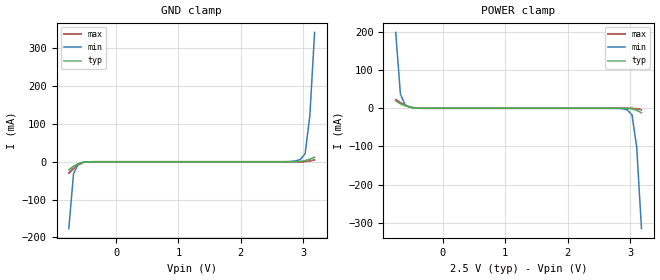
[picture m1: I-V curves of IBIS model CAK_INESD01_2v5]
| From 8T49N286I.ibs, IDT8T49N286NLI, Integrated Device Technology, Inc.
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| 4.00000e+00   -1.39435e-02   -4.76170e-01   -2.47919e-03
| 4.10000e+00   -3.14988e-02   -7.57889e-01   -1.14633e-02
| 4.20000e+00   -2.28002e-01   -1.04024e+00   -2.64916e-02
| 4.30000e+00   -6.05524e-01   -1.32301e+00   -4.21848e-02
| 4.40000e+00   -9.83643e-01   -1.60614e+00   -8.92880e-02
| 4.50000e+00   -1.36229e+00   -1.88958e+00   -5.31426e-01
| 4.60000e+00   -1.74142e+00   -2.17332e+00   -1.01589e+00
| 4.70000e+00   -2.12097e+00   -2.45733e+00   -1.50090e+00
| 4.80000e+00   -2.50090e+00   -2.74162e+00   -1.98635e+00
| 4.90000e+00   -2.88116e+00   -3.02615e+00   -2.47218e+00
| 5.00000e+00   -3.26171e+00   -3.31092e+00   -2.95830e+00
| 5.10000e+00   -3.64251e+00   -3.59590e+00   -3.44467e+00
| 5.20000e+00   -4.02353e+00   -3.88109e+00   -3.93123e+00
| 5.30000e+00   -4.40474e+00   -4.16647e+00   -4.41796e+00
| 5.40000e+00   -4.78610e+00   -4.45202e+00   -4.90484e+00
| 5.50000e+00   -5.16760e+00   -4.73774e+00   -5.39184e+00
| 5.60000e+00   -5.54921e+00   -5.02360e+00   -5.87893e+00
| 5.70000e+00   -5.93093e+00   -5.30959e+00   -6.36610e+00
| 5.80000e+00   -6.31272e+00   -5.59572e+00   -6.85331e+00
| 5.90000e+00   -6.69459e+00   -5.88196e+00   -7.34056e+00
| 6.00000e+00   -7.07651e+00   -6.16831e+00   -7.82783e+00
| 6.10000e+00   -7.45848e+00   -6.45476e+00   -8.31510e+00
| 6.20000e+00   -7.84049e+00   -6.74131e+00   -8.80238e+00
| 6.30000e+00   -8.22253e+00   -7.02794e+00   -9.28965e+00
| 6.40000e+00   -8.60459e+00   -7.31465e+00   -9.77691e+00
| 6.50000e+00   -8.98667e+00   -7.60144e+00   -1.02642e+01
| 6.60000e+00   -9.36876e+00   -7.88830e+00   -1.07514e+01
[Model]   CAK_INESD01_2v5
Model_type   Input
Polarity   Non-Inverting
Vinl = 0.7V
Vinh = 1.7V
|   typ   min   max
C_comp   2pF   1.5pF   2.5pF
|   typ   min   max
[Voltage range]   2.5V   2.375V   2.625V
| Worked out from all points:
|   GND clamp passes 1 mA (typ) near -0.50 V on its own axis
|   POWER clamp passes 1 mA (typ) near -0.46 V on its own axis
[GND_clamp]
|Voltage   I (typ)   I (min)   I (max)
|Note, modeling breaks down at 250mA and above.  This is well beyond the functional   |
|operating range of the device.  Should this scenario occur, catastrophic failure and   |
|possible damage to the device and/or board is of higher concern than the I-V curve   |
|behavior.  The IBIS checker will flag currents in excess of 10A with warnings.  Lines   |
|with currents in excess of 0.35 A have been commented out.  The points still remain|
|available to the user if the user desires to use them.   |
|-2.50000e+00   -6.31272e+00   -5.12654e+00   -7.65728e+00
|-2.42424e+00   -6.02348e+00   -4.90993e+00   -7.28814e+00
|-2.34848e+00   -5.73428e+00   -4.69340e+00   -6.91901e+00
|-2.27273e+00   -5.44513e+00   -4.47695e+00   -6.54991e+00
|-2.19697e+00   -5.15604e+00   -4.26060e+00   -6.18082e+00
|-2.12121e+00   -4.86701e+00   -4.04434e+00   -5.81177e+00
|-2.04545e+00   -4.57807e+00   -3.82819e+00   -5.44276e+00
|-1.96970e+00   -4.28920e+00   -3.61215e+00   -5.07380e+00
|-1.89394e+00   -4.00043e+00   -3.39622e+00   -4.70491e+00
|-1.81818e+00   -3.71177e+00   -3.18041e+00   -4.33609e+00
|-1.74242e+00   -3.42324e+00   -2.96474e+00   -3.96736e+00
|-1.66667e+00   -3.13483e+00   -2.74920e+00   -3.59872e+00
|-1.59091e+00   -2.84658e+00   -2.53381e+00   -3.23020e+00
|-1.51515e+00   -2.55849e+00   -2.31856e+00   -2.86179e+00
|-1.43939e+00   -2.27059e+00   -2.10347e+00   -2.49353e+00
|-1.36364e+00   -1.98290e+00   -1.88855e+00   -2.12544e+00
|-1.28788e+00   -1.69544e+00   -1.67379e+00   -1.75755e+00
|-1.21212e+00   -1.40822e+00   -1.45921e+00   -1.38989e+00
|-1.13636e+00   -1.12128e+00   -1.24483e+00   -1.02250e+00
|-1.06061e+00   -8.34620e-01   -1.03065e+00   -6.55423e-01
|-9.84848e-01   -5.48283e-01   -8.16712e-01   -2.88690e-01
|-9.09091e-01   -2.62296e-01   -6.03100e-01   -6.18054e-02
|-8.33333e-01   -5.02557e-02   -3.89957e-01   -4.19365e-02
-757.6mV  -21.75mA   -176.8mA   -30.27mA
-681.8mV  -11.92mA   -31.42mA   -17.96mA
-606.1mV  -5.225mA   -6.638mA   -8.107mA
-530.3mV  -1.487mA   -1.607mA   -2.246mA
-378.8mV  -25.75uA   -53.93uA   -24.13uA
2.727V    375.4nA    100.9uA    84.96pA
2.879V    106.8uA    2.187mA    552.6nA
2.955V    792.8uA    6.111mA    14.78uA
3.03V     2.866mA    21.14mA    228.9uA
3.106V    6.546mA    121.9mA    1.635mA
3.182V    11.87mA    341.6mA    5.025mA
| 3.25758e+00   1.96321e-02   5.60094e-01   1.03978e-02
| 3.33333e+00   4.87341e-02   7.78554e-01   1.76586e-02
| 3.40909e+00   2.77089e-01   9.97183e-01   2.56603e-02
| 3.48485e+00   5.68769e-01   1.21602e+00   3.28270e-02
| 3.56061e+00   8.60711e-01   1.43506e+00   7.83184e-02
| 3.63636e+00   1.15294e+00   1.65432e+00   4.20952e-01
| 3.71212e+00   1.44546e+00   1.87380e+00   7.94407e-01
| 3.78788e+00   1.73826e+00   2.09348e+00   1.16822e+00
| 3.86364e+00   2.03134e+00   2.31338e+00   1.54240e+00
| 3.93939e+00   2.32470e+00   2.53350e+00   1.91692e+00
| 4.01515e+00   2.61833e+00   2.75382e+00   2.29178e+00
| 4.09091e+00   2.91222e+00   2.97435e+00   2.66697e+00
| 4.16667e+00   3.20638e+00   3.19510e+00   3.04248e+00
| 4.24242e+00   3.50078e+00   3.41605e+00   3.41830e+00
| 4.31818e+00   3.79544e+00   3.63722e+00   3.79442e+00
| 4.39394e+00   4.09035e+00   3.85860e+00   4.17082e+00
| 4.46970e+00   4.38551e+00   4.08019e+00   4.54751e+00
| 4.54545e+00   4.68090e+00   4.30200e+00   4.92447e+00
| 4.62121e+00   4.97653e+00   4.52403e+00   5.30170e+00
| 4.69697e+00   5.27241e+00   4.74629e+00   5.67919e+00
| 4.77273e+00   5.56852e+00   4.96876e+00   6.05694e+00
| 4.84848e+00   5.86487e+00   5.19147e+00   6.43493e+00
| 4.92424e+00   6.16146e+00   5.41442e+00   6.81318e+00
| 5.00000e+00   6.45829e+00   5.63760e+00   7.19167e+00
[Power_clamp]
|Voltage   I (typ)   I (min)   I (max)
|Note, modeling breaks down at 250mA and above.  This is well beyond the functional   |
|operating range of the device.  Should this scenario occur, catastrophic failure and   |
|possible damage to the device and/or board is of higher concern than the I-V curve   |
|behavior.  The IBIS checker will flag currents in excess of 10A with warnings.  Lines   |
|with currents in excess of 0.35 A have been commented out.  The points still remain|
|available to the user if the user desires to use them.   |
|-2.50000e+00   6.45829e+00   5.26948e+00   7.81670e+00
|-2.42424e+00   6.16146e+00   5.04669e+00   7.43781e+00
|-2.34848e+00   5.86487e+00   4.82413e+00   7.05917e+00
|-2.27273e+00   5.56852e+00   4.60180e+00   6.68076e+00
|-2.19697e+00   5.27241e+00   4.37969e+00   6.30261e+00
|-2.12121e+00   4.97653e+00   4.15780e+00   5.92470e+00
|-2.04545e+00   4.68090e+00   3.93613e+00   5.54704e+00
|-1.96970e+00   4.38551e+00   3.71468e+00   5.16964e+00
|-1.89394e+00   4.09035e+00   3.49344e+00   4.79251e+00
|-1.81818e+00   3.79544e+00   3.27241e+00   4.41564e+00
|-1.74242e+00   3.50078e+00   3.05159e+00   4.03905e+00
|-1.66667e+00   3.20638e+00   2.83098e+00   3.66274e+00
|-1.59091e+00   2.91222e+00   2.61058e+00   3.28673e+00
|-1.51515e+00   2.61833e+00   2.39040e+00   2.91102e+00
|-1.43939e+00   2.32470e+00   2.17042e+00   2.53562e+00
|-1.36364e+00   2.03134e+00   1.95066e+00   2.16054e+00
|-1.28788e+00   1.73826e+00   1.73111e+00   1.78580e+00
|-1.21212e+00   1.44546e+00   1.51178e+00   1.41140e+00
|-1.13636e+00   1.15294e+00   1.29266e+00   1.03735e+00
|-1.06061e+00   8.60711e-01   1.07375e+00   6.63656e-01
|-9.84848e-01   5.68769e-01   8.55052e-01   2.90327e-01
|-9.09091e-01   2.77089e-01   6.36541e-01   4.67878e-02
|-8.33333e-01   4.87341e-02   4.18109e-01   3.00573e-02
-757.6mV  19.63mA    199mA      22.98mA
-681.8mV  11.87mA    37mA       14.92mA
-606.1mV  6.546mA    8.97mA     8.294mA
-530.3mV  2.866mA    3.16mA     3.61mA
-303mV    8.428uA    25.32uA    5.206uA
2.803V    -1.864uA   -178.3uA   -2.484nA
2.955V    -244.9uA   -4.054mA   -3.17uA
3.03V     -1.487mA   -17.6mA    -63.94uA
3.106V    -5.225mA   -102.4mA   -675.5uA
3.182V    -11.92mA   -315.5mA   -3.788mA
